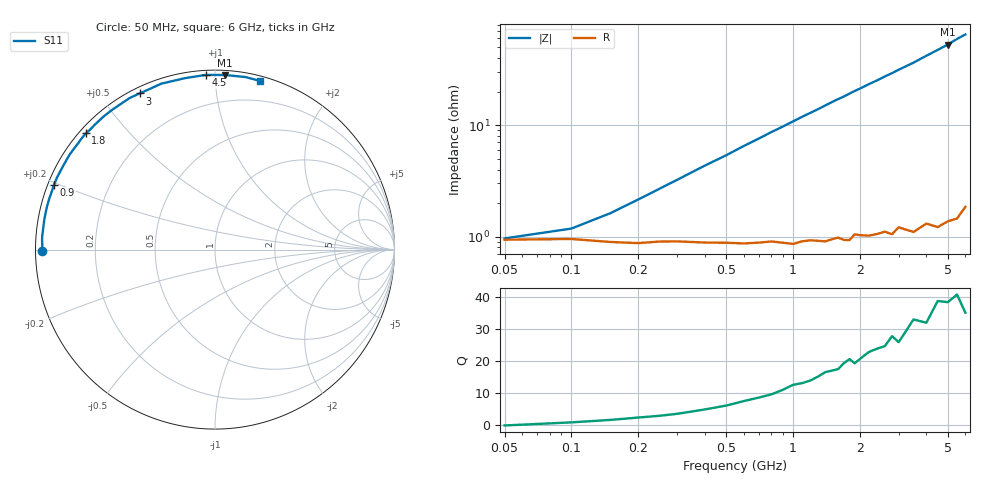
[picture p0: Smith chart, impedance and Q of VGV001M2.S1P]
! Infineon Technologies  Discrete & RF Semiconductors
! BB 831
! Si Tuning Diode in SOD323
! VR =
! S-Parameters:  July  1999
# GHz  S  MA  R  50
!  f  S11
! GHz  MAG  ANG
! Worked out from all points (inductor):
!   34 points, 50 MHz to 6 GHz, reference 50 ohm
!   read as one part to ground: L = 1.69 nH near 300 MHz
!   highest Q = 38.9 at 5 GHz (marker M1), where L = 1.68 nH
!   S11 on the Smith chart (normalised r, x): 50 MHz: 0.02, -0.00; 900 MHz: 0.02, +0.19; 1.8 GHz: 0.02, +0.38; 3 GHz: 0.02, +0.63; 4.5 GHz: 0.02, +0.95; 6 GHz: 0.04, +1.30
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0.05  0.9632 -179.5
0.1  0.9626 178.4
0.2  0.9657 175.5
0.4  0.9655 170.3
0.5  0.9657 167.9
0.6  0.9664 165.3
0.8  0.9655 160.4
0.9  0.9666 158.1
1  0.9677 155.7
1.1  0.9662 153.3
1.3  0.9665 148.9
1.5  0.9663 144.3
1.6  0.9656 142.2
1.7  0.9675 140.2
1.8  0.9681 138.0
1.9  0.9646 135.9
2  0.9657 134.0
2.2  0.967 130.0
2.4  0.9669 126.4
2.6  0.9665 122.6
2.8  0.9692 119.3
3  0.9658 115.7
3.5  0.9717 107.9
4  0.9697 100.0
4.5  0.9747 93.1
5  0.9744 86.8
5.5  0.9762 80.1
6  0.9729 75.0
